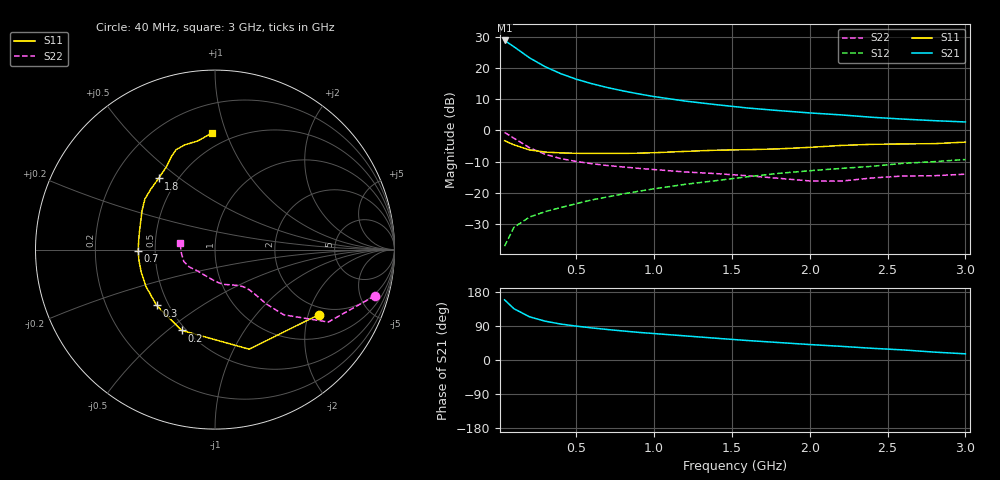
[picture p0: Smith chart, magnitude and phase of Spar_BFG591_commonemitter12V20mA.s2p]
! Filename:  BFG591B.S2P  Version:  4.0
! NXP part #: BFG591  Date: Jun 1994
! Bias condition: Vce=12V; Ic=20mA
#  MHz  S  MA  R  50
! Freq  S11  S21  S12  S22  !GUM [dB]
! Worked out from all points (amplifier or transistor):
!   21 points, 40 MHz to 3 GHz, reference 50 ohm
!   highest |S21| = 28.8 dB at 40 MHz (marker M1)
!   |S21| within 3 dB of that: start of sweep to 127.8 MHz
!   unconditionally stable (mu >= 1): 701.4 MHz to 2.191 GHz
!   at 300 MHz: K = 0.71, MSG = 23.2 dB, |S12| = -26.0 dB
!   at 1 GHz: K = 1.06, MAG = 13.3 dB, |S12| = -18.7 dB
!   at 3 GHz: K = 0.95, MSG = 6.0 dB, |S12| = -9.3 dB
!   S11 on the Smith chart (normalised r, x): 40 MHz: 1.73, -2.35; 200 MHz: 0.47, -0.56; 300 MHz: 0.43, -0.34; 700 MHz: 0.40, -0.01; 1.8 GHz: 0.39, +0.42; 3 GHz: 0.40, +0.89
40  0.683 -32.0  27.55 158.7  0.014 75.1  0.928 -16.1
100  0.587 -71.0  21.85 135.3  0.028 62.6  0.749 -32.6
200  0.487 -112.4  14.52 114.0  0.041 55.9  0.528 -43.5
300  0.45 -136.3  10.48 102.5  0.05 56.1  0.415 -46.7
400  0.436 -151.9  8.113 94.9  0.058 58.1  0.354 -47.7
500  0.43 -163.0  6.606 89.4  0.067 60.2  0.318 -48.6
600  0.428 -171.9  5.598 84.7  0.077 61.7  0.293 -49.6
700  0.428 -179.3  4.855 80.5  0.086 63.1  0.274 -51.0
800  0.428 173.8  4.294 76.6  0.096 63.9  0.26 -52.8
900  0.432 167.3  3.845 72.9  0.106 64.7  0.247 -55.1
1000  0.439 161.4  3.48 69.8  0.116 65.1  0.236 -57.9
1200  0.461 151.8  2.948 63.6  0.137 65.1  0.216 -65.2
1400  0.482 144.1  2.581 57.4  0.157 64.3  0.203 -73.6
1600  0.491 136.9  2.285 51.4  0.181 64.2  0.188 -82.6
1800  0.506 128.4  2.077 46.1  0.205 61.7  0.171 -93.0
2000  0.535 120.3  1.904 40.8  0.226 60.6  0.155 -109.9
2200  0.574 114.9  1.772 36.1  0.246 58.8  0.154 -129.9
2400  0.598 111.1  1.622 30.9  0.266 58.3  0.173 -146.1
2600  0.607 106.1  1.517 26.6  0.297 54.9  0.186 -159.0
2800  0.613 99.1  1.431 20.8  0.316 51.0  0.188 -173.1
3000  0.649 91.5  1.365 16.3  0.342 49.8  0.199 168.7
